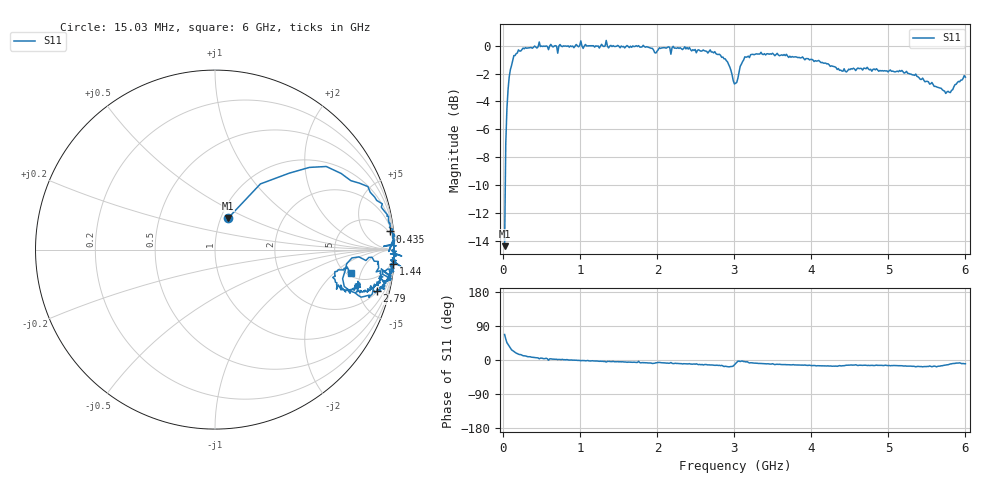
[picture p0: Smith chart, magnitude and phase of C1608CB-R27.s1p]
!	Network	Analyzer	HP8753E.07.74:	Oct	30	2002	Serial	No.	JP38451487
!	Hewlett-Packard
!	28	Aug	2009	8:35:38
!	Frequency	S11
#	HZ	S	RI	R	50
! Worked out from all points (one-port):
!   400 points, 15.03 MHz to 6 GHz, reference 50 ohm
!   lowest |S11| = -14.4 dB at 15.03 MHz (marker M1), VSWR 1.47, Z = 54.2 + j19.8 ohm
!   |S11| at or under -10 dB: start of sweep to 23.98 MHz
!   S11 on the Smith chart (normalised r, x): 15.03 MHz: 1.08, +0.40; 435 MHz: 3, +19; 1.44 GHz: 2, -25; 2.79 GHz: 2.11, -7.29; 6 GHz: 5.40, -3.52
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1.502992e7  0.0737 0.176
3.002985e7  0.253 0.366
4.502978e7  0.414 0.426
9.002955e7  0.703 0.424
1.350293e8  0.852 0.351
2.550287e8  0.962 0.192
4.350278e8  0.976 0.101
4.650277e8  1.03 0.0563
5.550272e8  0.995 0.0806
5.850271e8  0.968 -0.0103
6.00027e8  0.996 0.0515
7.050265e8  0.94 0.0186
7.650262e8  0.992 0.0301
1.440023e9  0.991 -0.079
1.515022e9  0.98 -0.0797
2.265019e9  0.972 -0.156
2.790016e9  0.901 -0.232
2.925015e9  0.814 -0.265
3.015015e9  0.724 -0.121
3.045015e9  0.763 -0.0464
3.135014e9  0.91 -0.0663
3.525012e9  0.9 -0.195
3.765011e9  0.89 -0.194
4.275009e9  0.81 -0.239
4.515007e9  0.806 -0.187
5.265004e9  0.763 -0.223
5.745001e9  0.656 -0.155
6e9  0.76 -0.132
